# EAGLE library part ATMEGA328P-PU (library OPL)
8-bit AVR Microcontroller with 32K Bytes In-System Programmable Flash
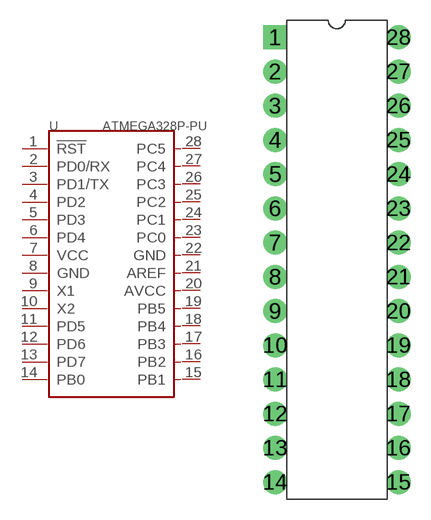
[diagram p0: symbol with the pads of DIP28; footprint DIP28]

Designator prefix U

## ATMEGA328P-PU-1030050P1  [DIP28]
1  !RST
2  PD0/RX
3  PD1/TX
4  PD2
5  PD3
6  PD4
7  VCC
8  GND
9  X1
10  X2
11  PD5
12  PD6
13  PD7
14  PB0
15  PB1
16  PB2
17  PB3
18  PB4
19  PB5
20  AVCC
21  AREF
22  GND
23  PC0
24  PC1
25  PC2
26  PC3
27  PC4
28  PC5

## Footprint DIP28 (pad centres in mm)
drill 1.016 pad 1.778 square: 1 -4.572,16.51
drill 1.016 pad 1.778: 2 -4.572,13.97; 3 -4.572,11.43; 4 -4.572,8.89; 5 -4.572,6.35; 6 -4.572,3.81; 7 -4.572,1.27; 8 -4.572,-1.27; 9 -4.572,-3.81; 10 -4.572,-6.35; 11 -4.572,-8.89; 12 -4.572,-11.43; 13 -4.572,-13.97; 14 -4.572,-16.51; 15 4.572,-16.51; 16 4.572,-13.97; 17 4.572,-11.43; 18 4.572,-8.89; 19 4.572,-6.35; 20 4.572,-3.81; 21 4.572,-1.27; 22 4.572,1.27; 23 4.572,3.81; 24 4.572,6.35; 25 4.572,8.89; 26 4.572,11.43; 27 4.572,13.97; 28 4.572,16.51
